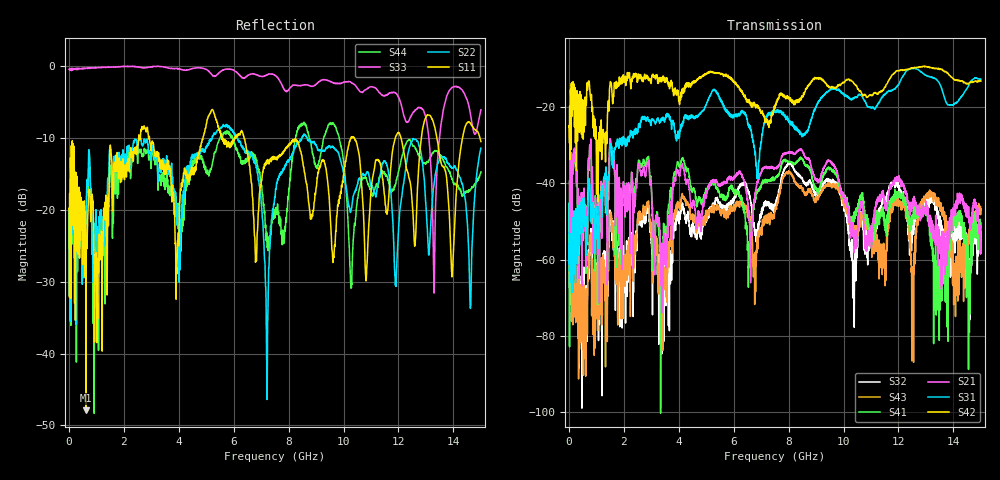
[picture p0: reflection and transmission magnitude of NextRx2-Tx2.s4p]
!  = SDD11
!  = SDD12
!  = SDC11
!  = SDC12
!  = SDD21
!  = SDD22
!  = SDC21
!  = SDC22
!  = SCD11
!  = SCD12
!  = SCC11
!  = SCC12
!  = SCD21
!  = SCD22
!  = SCC21
!  = SCC22
! FILE: N:\QM 2007\Prüfprotokolle\Highspeed\Konfektionierte Ltg\L45593-D106\D30\8216\0002\Next\NextRx2-Tx2.s4p
# MHz S DB R 50.00
! FREQ  S11  S12  S13  S14
!  S21  S22  S23  S24
!  S31  S32  S33  S34
!  S41  S42  S43  S44
!  DB  ANG  DB  ANG  DB  ANG  DB  ANG
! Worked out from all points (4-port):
!   2999 points, 10 MHz to 15 GHz, reference 50 ohm
!   strongest paths, dB at 10 MHz, 3.755 GHz, 7.505 GHz, 11.26 GHz, 15 GHz:
!     S42: -25.2, -13.5, -20.0, -16.6, -13.2
!     S31: -45.3, -24.2, -21.1, -19.1, -12.7
!     S21: -52.8, -47.8, -36.1, -44.1, -55.5
!     S41: -52.8, -46.2, -38.6, -47.8, -52.8
!     S43: -49.4, -56.3, -47.1, -58.5, -47.0
!     S32: -52.7, -60.4, -46.3, -48.0, -52.9
!   lowest |S11| = -47.9 dB at 625 MHz (marker M1), VSWR 1.01, Z = 50 + j0.402 ohm
!   |S11| at or under -10 dB: start of sweep to 2.54 GHz; 2.936 GHz to 4.884 GHz (1.948 GHz wide, 49.8 % of centre); 6.376 GHz to 10.27 GHz (3.895 GHz wide, 46.8 % of centre)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
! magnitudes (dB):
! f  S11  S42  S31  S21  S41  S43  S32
! 10 MHz  -19.8  -25.2  -45.3  -52.8  -52.8  -49.4  -52.7
! 625 MHz  -47.9  -17.4  -49.9  -53.0  -53.5  -70.4  -66.8
! 5.79 GHz  -11.1  -11.6  -21.1  -39.1  -42.5  -47.6  -45.7
! 7.215 GHz  -13.4  -23.9  -22.1  -35.9  -39.6  -49.8  -45.7
! 8.03 GHz  -10.9  -17.5  -23.7  -31.9  -34.3  -37.2  -34.7
! 10.39 GHz  -10.0  -14.0  -17.7  -56.6  -48.5  -51.9  -68.7
! 15 GHz  -10.5  -13.2  -12.7  -55.5  -52.8  -47.0  -52.9
